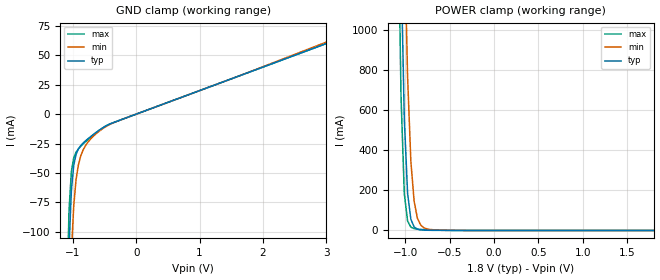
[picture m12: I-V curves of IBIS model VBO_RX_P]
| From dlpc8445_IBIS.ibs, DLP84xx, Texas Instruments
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|   Model VBO_RX_P
[Model] VBO_RX_P
Model_type Input
Polarity   Non-Inverting
Enable   Active-High
Vinl =  -5.000mV
Vinh =  5.000mV
C_comp   0.805pF   0.728pF   0.884pF
C_comp_power_clamp   0.0F   1.29fF   2.289fF
[Model Spec]
Vinh   5.000mV   5.000mV   5.000mV
Vinl   -5.000mV   -5.000mV   -5.000mV
[Temperature Range]   25.000   0.125k   -40.000
[Voltage Range]   1.800V   1.620V   1.980V
[POWER Clamp Reference]   1.800V   1.620V   1.980V
[GND Clamp Reference]   0.0V   0.0V   0.0V
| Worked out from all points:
|   GND clamp passes 1 mA (typ) near -0.05 V on its own axis
|   POWER clamp passes 1 mA (typ) near -0.72 V on its own axis
[GND_clamp]
|Voltage   I(typ)   I(min)   I(max)
-1.8V     -6.93A     -6.979A    -7.166A
-1.097V   -211.3mA   -301.9mA   -165.8mA
-1.06V    -114mA     -189.3mA   -81.79mA
-1.023V   -65.2mA    -118.8mA   -48.92mA
-986mV    -43.66mA   -78.24mA   -37.29mA
-949mV    -34.21mA   -55.77mA   -32.44mA
-912mV    -29.54mA   -43.12mA   -29.61mA
-875mV    -26.71mA   -35.52mA   -27.4mA
-801mV    -22.74mA   -26.88mA   -23.55mA
-727mV    -19.42mA   -21.59mA   -20.02mA
-505mV    -10.93mA   -11.52mA   -10.87mA
3.6V      72.09mA    73.82mA    72.04mA
[POWER_clamp]
|Voltage   I(typ)   I(min)   I(max)
-1.789V   24.16A     24.62A     27.1A
-1.086V   2.583A     3.93A      1.733A
-1.049V   1.355A     2.601A     671.3mA
-1.012V   557.6mA    1.517A     184.5mA
-975mV    185.7mA    768.4mA    47.38mA
-938mV    56.22mA    345.3mA    16.71mA
-901mV    17.43mA    145.3mA    9.302mA
-864mV    6.234mA    60.79mA    6.7mA
-827mV    2.874mA    26.76mA    5.227mA
-753mV    1.224mA    7.312mA    3.286mA
-346mV    65.21uA    300.5uA    163.8uA
1.8V      0A         0A         0A
